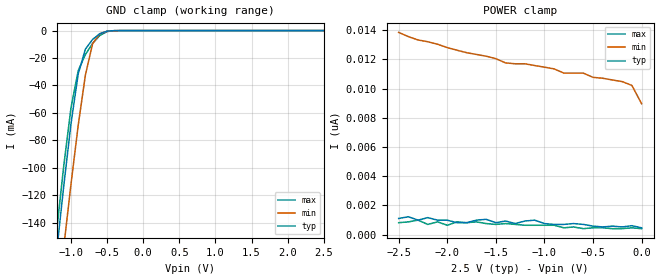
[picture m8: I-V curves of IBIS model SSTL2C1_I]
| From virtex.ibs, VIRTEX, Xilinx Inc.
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|   Model SSTL2C1_I
[Model]   SSTL2C1_I
Model_type   Input
Polarity   Non-Inverting
Vinl =   1.070V
Vinh =   1.430V
C_comp   6.5000pF   5.0000pF   8.0000pF
[Temperature Range]   27.0000   100.0000   0.000
[Voltage Range]   2.5000V   2.3750V   2.6250V
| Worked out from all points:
|   GND clamp passes 1 mA (typ) near -0.53 V on its own axis
[GND_clamp]
| voltage   I(typ)   I(min)   I(max)
-2.5V     -851.8mA   -860.9mA   -847.5mA
-1.2V     -161.8mA   -205.3mA   -146.7mA
-1.1V     -113.2mA   -157.8mA   -98.56mA
-1V       -68.04mA   -112mA     -56.27mA
-900mV    -31.6mA    -69.09mA   -29.2mA
-800mV    -13.5mA    -32.34mA   -17.42mA
-700mV    -6.408mA   -9.455mA   -9.303mA
-600mV    -2.237mA   -2.349mA   -3.538mA
-500mV    -423.5uA   -545.3uA   -698.2uA
-400mV    -42.44uA   -91.28uA   -59.93uA
2.5V      465.7pA    32.48nA    261.9pA
[POWER_clamp]
| voltage   I(typ)   I(min)   I(max)
-2.5V     1.106nA    13.85nA    814.9pA
-2.4V     1.222nA    13.56nA    873.1pA
-2.3V     989.5pA    13.33nA    989.5pA
-2.2V     1.164nA    13.21nA    698.5pA
-2.1V     989.5pA    13.04nA    873.1pA
-2V       989.5pA    12.81nA    640.3pA
-1.9V     814.9pA    12.63nA    873.1pA
-1.6V     1.048nA    12.22nA    756.7pA
-1.4V     931.3pA    11.76nA    756.7pA
-200mV    523.9pA    10.48nA    407.5pA
-100mV    611.2pA    10.22nA    465.7pA
0V        465.7pA    8.964nA    407.5pA
